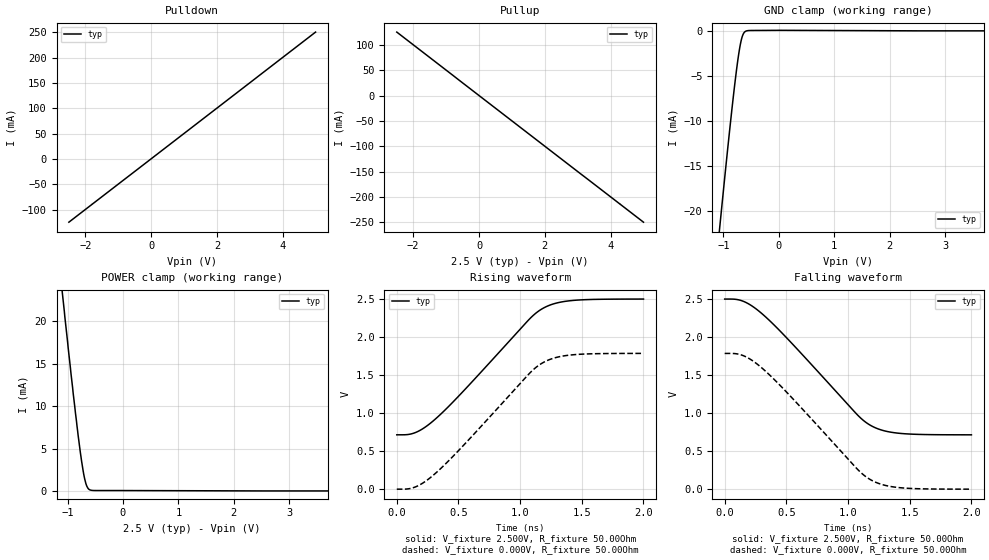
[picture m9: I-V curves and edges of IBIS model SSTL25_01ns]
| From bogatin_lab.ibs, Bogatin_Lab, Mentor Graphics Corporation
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[Model]   SSTL25_01ns
Model_type   I/O
Vinl = 800.000mV
Vinh = 2.000V
Vmeas = 1.500V
Vref = 0.000V
Cref = 50.000pF
Rref = 1.000kOhm
|   typ   min   max
C_comp   4.000pF   NA   NA
[Voltage Range]   2.500V   NA   NA
[Temperature Range]   50.0   NA   NA
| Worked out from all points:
|   slope of the pulldown table from 0 to 0.375 V, typ, clamps not added: 20 ohm
|   slope of the pullup table from 0 to 0.375 V, typ, clamps not added: 20 ohm
|   GND clamp passes 1 mA (typ) near -0.68 V on its own axis
|   POWER clamp passes 1 mA (typ) near -0.68 V on its own axis
|   falling waveform, V_fixture 2.500V, R_fixture 50.00Ohm: 20-80 % time 612ps typ, NA min, NA max; typ from 2.5 V to 0.712 V
|   rising waveform, V_fixture 2.500V, R_fixture 50.00Ohm: 20-80 % time 612ps typ, NA min, NA max; typ from 0.712 V to 2.5 V
|   rising waveform, V_fixture 0.000V, R_fixture 50.00Ohm: 20-80 % time 612ps typ, NA min, NA max; typ from -0.002 V to 1.78 V
|   falling waveform, V_fixture 0.000V, R_fixture 50.00Ohm: 20-80 % time 612ps typ, NA min, NA max; typ from 1.78 V to -0.002 V
[Pulldown]
|   Voltage   I(typ)   I(min)   I(max)
-2.5V     -124.8mA   NA         NA
-1.79V    -88.98mA   NA         NA
-1.78V    -88.92mA   NA         NA
5V        250.1mA    NA         NA
[GND Clamp]
|   Voltage   I(typ)   I(min)   I(max)
-2.5V     -114.3mA   NA         NA
-1.09V    -23.21mA   NA         NA
-1.05V    -20.74mA   NA         NA
-930mV    -13.48mA   NA         NA
-850mV    -8.858mA   NA         NA
-790mV    -5.639mA   NA         NA
-740mV    -3.241mA   NA         NA
-700mV    -1.682mA   NA         NA
-670mV    -832.5uA   NA         NA
-640mV    -324.9uA   NA         NA
-600mV    -49.63uA   NA         NA
5V        0A         NA         NA
[Pullup]
|   Voltage   I(typ)   I(min)   I(max)
-2.5V     125.3mA    NA         NA
4.28V     -213.8mA   NA         NA
4.29V     -213.7mA   NA         NA
5V        -249.7mA   NA         NA
[POWER Clamp]
|   Voltage   I(typ)   I(min)   I(max)
-2.5V     114.2mA    NA         NA
-1.11V    24.28mA    NA         NA
-1.08V    22.46mA    NA         NA
-990mV    16.9mA     NA         NA
-900mV    11.56mA    NA         NA
-810mV    6.552mA    NA         NA
-750mV    3.619mA    NA         NA
-710mV    2.012mA    NA         NA
-670mV    864.1uA    NA         NA
-630mV    292.7uA    NA         NA
-600mV    133.4uA    NA         NA
5V        0A         NA         NA
[Ramp]
R_load = 50.00Ohm
|   typ   min   max
dV/dt_r   1.071V/611.703ps   NA   NA
dV/dt_f   1.071V/611.703ps   NA   NA
[Falling Waveform]
V_fixture = 2.500V
R_fixture = 50.00Ohm
|   Time   V(typ)   V(min)   V(max)
0s        2.497V     NA         NA
150.5ps   2.468V     NA         NA
222.9ps   2.404V     NA         NA
305ps     2.301V     NA         NA
531.8ps   1.937V     NA         NA
1.077ns   972.6mV    NA         NA
1.189ns   830.9mV    NA         NA
1.292ns   765.8mV    NA         NA
1.427ns   730.6mV    NA         NA
2ns       712.3mV    NA         NA
[Rising Waveform]
V_fixture = 2.500V
R_fixture = 50.00Ohm
|   Time   V(typ)   V(min)   V(max)
0s        712.3mV    NA         NA
150.5ps   741.9mV    NA         NA
222.9ps   805.4mV    NA         NA
305ps     908.8mV    NA         NA
531.8ps   1.273V     NA         NA
1.077ns   2.237V     NA         NA
1.189ns   2.379V     NA         NA
1.292ns   2.444V     NA         NA
1.427ns   2.479V     NA         NA
2ns       2.497V     NA         NA
[Rising Waveform]
V_fixture = 0.000V
R_fixture = 50.00Ohm
|   Time   V(typ)   V(min)   V(max)
0s        -2.067mV   NA         NA
150.5ps   27.18mV    NA         NA
222.9ps   90.66mV    NA         NA
305ps     194.1mV    NA         NA
529.9ps   555mV      NA         NA
1.077ns   1.523V     NA         NA
1.189ns   1.664V     NA         NA
1.292ns   1.729V     NA         NA
1.429ns   1.765V     NA         NA
2ns       1.783V     NA         NA
[Falling Waveform]
V_fixture = 0.000V
R_fixture = 50.00Ohm
|   Time   V(typ)   V(min)   V(max)
0s        1.783V     NA         NA
150.5ps   1.753V     NA         NA
222.9ps   1.69V      NA         NA
305ps     1.586V     NA         NA
531.8ps   1.222V     NA         NA
1.077ns   258.2mV    NA         NA
1.189ns   116.5mV    NA         NA
1.292ns   51.39mV    NA         NA
1.427ns   16.26mV    NA         NA
2ns       -2.067mV   NA         NA
